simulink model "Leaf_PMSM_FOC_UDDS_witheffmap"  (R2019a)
settings: Solver=VariableStepAuto  StartTime=0.0  StopTime=764  FixedStep=1e-3  MaxStep=1e-3  RelTol=1e-3
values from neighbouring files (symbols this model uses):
  B = 0    [PMSM_EV_init_v2.m]    (also in Leaf_Initialization.m; Tesla_Initialization.m)
  Eoff = 201e-6    (= 0.000201)    [DeviceParam.m]
  Eoff_diode = 1.4e-3    (= 0.0014)    [DeviceParam.m]
  Eoff_Si = 2.15e-3    (= 0.00215)    [DeviceParam.m]
  Eon = 252e-6    (= 0.000252)    [DeviceParam.m]
  Eon_Si = 1.2e-3    (= 0.0012)    [DeviceParam.m]
  fs = 10000    [PMSM_EV_init_v2.m]    (also in Leaf_Initialization.m; Tesla_Initialization.m)
  I_DS_data = [-36 36 62]    [DeviceParam.m]
  IC_data = [0 30 60]    [DeviceParam.m]
  Inom = 75    [DeviceParam.m]    (also in Iqbal Husain - Example12_1.m = Psm/VsmNom)
  J = 0.3    [PMSM_EV_init_v2.m]    (also in Leaf_Initialization.m; Tesla_Initialization.m)
  Leaf_id_axis = [-2.296328E+02	-2.041181E+02	-1.786033E+02	-1.530886E+02	-1.275738E+02	-1.020590E+02	-7.654428E+01	-5.102952E+01	-2.551476E+01	+0.000000E+00]    [Leaf_Param.m]    (also in Leaf_Initialization.m)
  Leaf_iq_axis = [+0.000000E+00	+2.551476E+01	+5.102952E+01	+7.654428E+01	+1.020590E+02	+1.275738E+02	+1.530886E+02	+1.786033E+02	+2.041181E+02	+2.296328E+02]    [Leaf_Param.m]    (also in Leaf_Initialization.m)
  Leaf_Ld = [+4.562516E-04	+4.676675E-04	+4.893199E-04	+5.037353E-04	+5.104223E-04	+5.166612E-04	+5.237499E-04	+5.295159E-04	+5.345150E-04	+5.371060E-04    [Leaf_Param.m]    (also in Leaf_Initialization.m)
  Leaf_Lq = [+1.028048E-03	+1.047482E-03	+1.072792E-03	+1.100303E-03	+1.125549E-03	+1.152180E-03	+1.181188E-03	+1.211466E-03	+1.243133E-03	+1.273628E-03    [Leaf_Param.m]    (also in Leaf_Initialization.m)
  Leaf_omega_axis = [+0.000000E+00	+3.935365E+01	+7.870730E+01	+1.180610E+02	+1.574146E+02	+1.967683E+02	+2.361219E+02	+2.754756E+02	+3.857216E+02	+4.959676E+02	+6.062136E+02	+7.164596E+02	+8.267056E+02	+9.369516E+02	+1.047198E+03]    [Leaf_Param.m]    (also in Leaf_Initialization.m)
  Leaf_phid = [-4.199708E-02	-2.553401E-02	-8.247090E-03	+9.778563E-03	+2.810579E-02	+4.661402E-02	+6.539149E-02	+8.441129E-02	+1.036049E-01	+1.229854E-01    [Leaf_Param.m]    (also in Leaf_Initialization.m)
  Leaf_phiq = [-1.952292E-05	-3.396145E-06	+2.962394E-07	-2.077424E-05	-3.654397E-05	-1.649631E-05	+3.339687E-05	+4.306712E-05	+9.669480E-06	-2.373166E-05    [Leaf_Param.m]    (also in Leaf_Initialization.m)
  Leaf_T = [-3.804040E-02	-5.882121E-03	+4.489506E-04	-2.698573E-02	-3.955883E-02	-1.428580E-02	+2.169126E-02	+1.864805E-02	+2.093441E-03	+0.000000E+00    [Leaf_Param.m]    (also in Leaf_Initialization.m)
  Leaf_torque_axis = [+0.000000E+00	+1.167089E+01	+2.334179E+01	+3.501268E+01	+4.668357E+01	+5.835446E+01	+7.002536E+01	+7.910792E+01	+9.076234E+01	+1.063042E+02	+1.281510E+02	+1.612785E+02	+2.121831E+02	+2.805757E+02]    [Leaf_Param.m]    (also in Leaf_Initialization.m)
  P = 8    [PMSM_EV_init_v2.m]    (also in Iqbal Husain - Example12_1.m = V.*I; Leaf_Initialization.m; Tesla_Initialization.m)
  Rd_IGBT = (1.4-0.9)/(60-15)    (= 0.0111111111111)    [DeviceParam.m]
  RDS_on_data = [25e-3 27e-3 28e-3]    [DeviceParam.m]
  Rs = 0.046    [PMSM_EV_init_v2.m]    (also in Leaf_Initialization.m; Tesla_Initialization.m)
  Speed = [+0.000000E+00	+6.054730E+02	+1.210946E+03	+1.816419E+03	+2.421892E+03	+3.027365E+03	+3.632838E+03	+4.238311E+03	+5.775695E+03	+7.313079E+03	+8.850463E+03	+1.038785E+04	+1.192523E+04	+1.346262E+04	+1.500000E+04]    [PMSM_EV_init_v2.m]
  Torque = [+0.000000E+00	+7.333624E+00	+1.466725E+01	+2.200087E+01	+2.933450E+01	+3.666812E+01	+4.400174E+01	+5.043561E+01	+5.870849E+01	+6.980054E+01	+8.566293E+01	+1.107686E+02	+1.535327E+02	+2.089386E+02]    [PMSM_EV_init_v2.m]
  Vbatt = Vdc    (= 375)    [PMSM_EV_init_v2.m]    (also in Leaf_Initialization.m; Tesla_Initialization.m)
  VCE_data = [0 1.1 1.45]    [DeviceParam.m]
  Vd_IGBT = 1.5    [DeviceParam.m]
  Vdc = 375    [PMSM_EV_init_v2.m]    (also in Leaf_Initialization.m; Tesla_Initialization.m)
  Vnom = 300    [DeviceParam.m]
undefined symbols (not defined in the file or in its folder): A1, B1370, B766, HEV_Param, plecs
libraries: fl_lib x18, nesl_utility x9, sdl_lib x4, powerlib_meascontrol x3
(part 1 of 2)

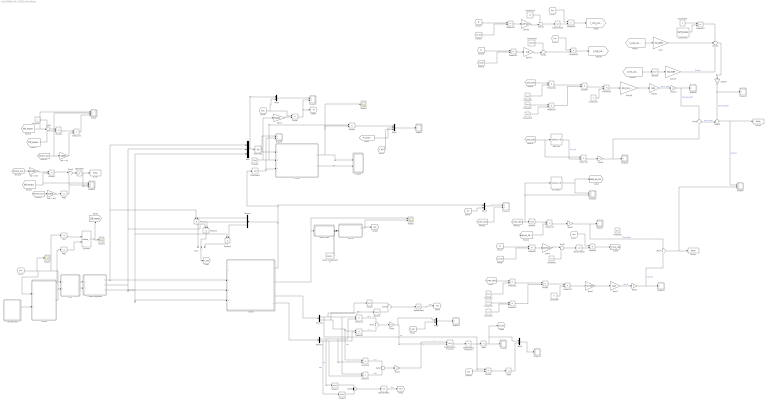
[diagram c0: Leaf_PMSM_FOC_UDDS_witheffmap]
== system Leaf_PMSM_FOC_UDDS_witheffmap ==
  Abs{,1..4} (5 alike) : Abs
  Circuit : Subsystem  LoadFcn=plecs('sl', 200);  InitFcn=plecs('sl', 214);  StartFcn=plecs('sl', 208);  StopFcn=plecs('sl', 209);  mask(PlecsCircuit){PLECSData=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}
      mask prompts: PLECSData "PLECS Data (Do not delete or modify!)"
      mask init:
      | % PLACE CUSTOM INITIALIZATIONS ABOVE
      | % DO NOT REMOVE
      | plecs('sl', 215);
      | % DO NOT REMOVE
  Constant : Constant  Value=Vbatt
  Constant1 : Constant  Value=1/8
  Constant10 : Constant  Value=Inom
  Constant11 : Constant  Value=fs
  Constant12 : Constant  Value=1/8
  Constant13 : Constant  Value=1/(2*pi)
  Constant14 : Constant  Value=fs
  Constant15 : Constant  Value=Eoff_diode
  Constant2 : Constant  Commented=on  Value=30e-3
  Constant3 : Constant  Value=Vbatt
  Constant4 : Constant  Value=Vnom
  Constant5 : Constant  Value=Inom
  Constant6 : Constant  Value=fs
  Constant7 : Constant
  Constant8 : Constant  Value=Vbatt
  Constant9 : Constant  Value=Vnom
  Control : Subsystem
  Current Regulator : Subsystem
  Currents : Subsystem  LoadFcn=plecs('sl', 300);  InitFcn=plecs('sl', 314);  StartFcn=plecs('sl', 308);  StopFcn=plecs('sl', 309);  mask{Settings=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}
      mask init:
      | plecs('sl', 315);
  Demux : Demux  Outputs=3
  Demux1 : Demux  Outputs=2
  Demux2 : Demux  Outputs=2
  Divide{,1..5} (6 alike) : Product  Inputs=*/
  FOC : Subsystem
  Gain : Gain  Gain=Vd_IGBT
  Gain1 : Gain  Gain=1.5
  Gain10 : Gain  Gain=Eon_Si+Eoff_Si
  Gain11 : Gain  Gain=1/pi
  Gain{5,8..9,12,16} (5 alike) : Gain  Gain=6
  Gain13 : Gain  Gain=1/(3*pi)
  Gain14 : Gain  Gain=1/8
  Gain15 : Gain  Gain=Rd_IGBT
  Gain2 : Gain  Gain=1.5
  Gain3 : Gain  Gain=1/sqrt(3)
  Gain4 : Gain  Gain=1/(3*pi)
  Gain6 : Gain  Gain=Eon+Eoff
  Gain7 : Gain  Gain=1/pi
  IGBT Vce : Lookup_n-D  NumberOfTableDimensions=1  BreakpointsForDimension1=IC_data  Table=VCE_data  InternalRulePriority=Speed  RndMeth=Simplest
  Iq_camry : Lookup_n-D  BreakpointsForDimension1=Leaf_omega_axis  BreakpointsForDimension2=Leaf_torque_axis  Table=Leaf_Eff'  InternalRulePriority=Speed  RndMeth=Simplest
  Kph demand : Subsystem
  Motor Shaft : Subsystem
  Mux : Mux  Inputs=3
  Mux1 : Mux  Inputs=3
  Mux{2..5} (4 alike) : Mux  Inputs=2
  PMSM : Subsystem
  Product{,1..23} (24 alike) : Product
  Saturation : Saturate  UpperLimit=10e3  LowerLimit=0
  Scope : Subsystem  LoadFcn=plecs('sl', 300);  InitFcn=plecs('sl', 314);  StartFcn=plecs('sl', 308);  StopFcn=plecs('sl', 309);  mask{Settings=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}
      mask init:
      | plecs('sl', 315);
  Scope1 : Scope
  Scope10 : Subsystem  LoadFcn=plecs('sl', 300);  InitFcn=plecs('sl', 314);  StartFcn=plecs('sl', 308);  StopFcn=plecs('sl', 309);  mask{Settings=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}
      mask init:
      | plecs('sl', 315);
  Scope11 : Subsystem  LoadFcn=plecs('sl', 300);  InitFcn=plecs('sl', 314);  StartFcn=plecs('sl', 308);  StopFcn=plecs('sl', 309);  mask{Settings=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}
      mask init:
      | plecs('sl', 315);
  Scope12 : Subsystem  LoadFcn=plecs('sl', 300);  InitFcn=plecs('sl', 314);  StartFcn=plecs('sl', 308);  StopFcn=plecs('sl', 309);  mask{Settings=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}
      mask init:
      | plecs('sl', 315);
  Scope13 : Subsystem  LoadFcn=plecs('sl', 300);  InitFcn=plecs('sl', 314);  StartFcn=plecs('sl', 308);  StopFcn=plecs('sl', 309);  mask{Settings=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}
      mask init:
      | plecs('sl', 315);
  Scope14 : Subsystem  LoadFcn=plecs('sl', 300);  InitFcn=plecs('sl', 314);  StartFcn=plecs('sl', 308);  StopFcn=plecs('sl', 309);  mask{Settings=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}
      mask init:
      | plecs('sl', 315);
  Scope15 : Subsystem  LoadFcn=plecs('sl', 300);  InitFcn=plecs('sl', 314);  StartFcn=plecs('sl', 308);  StopFcn=plecs('sl', 309);  mask{Settings=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}
      mask init:
      | plecs('sl', 315);
  Scope16 : Subsystem  LoadFcn=plecs('sl', 300);  InitFcn=plecs('sl', 314);  StartFcn=plecs('sl', 308);  StopFcn=plecs('sl', 309);  mask{Settings=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}
      mask init:
      | plecs('sl', 315);
  Scope17 : Subsystem  LoadFcn=plecs('sl', 300);  InitFcn=plecs('sl', 314);  StartFcn=plecs('sl', 308);  StopFcn=plecs('sl', 309);  mask{Settings=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}
      mask init:
      | plecs('sl', 315);
  Scope18 : Subsystem  LoadFcn=plecs('sl', 300);  InitFcn=plecs('sl', 314);  StartFcn=plecs('sl', 308);  StopFcn=plecs('sl', 309);  mask{Settings=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}
      mask init:
      | plecs('sl', 315);
  Scope19 : Subsystem  LoadFcn=plecs('sl', 300);  InitFcn=plecs('sl', 314);  StartFcn=plecs('sl', 308);  StopFcn=plecs('sl', 309);  mask{Settings=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}
      mask init:
      | plecs('sl', 315);
  Scope2 : Scope  NumInputPorts=2
  Scope3 : Scope
  Scope4 : Subsystem  LoadFcn=plecs('sl', 300);  InitFcn=plecs('sl', 314);  StartFcn=plecs('sl', 308);  StopFcn=plecs('sl', 309);  mask{Settings=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}
      mask init:
      | plecs('sl', 315);
  Scope5 : Subsystem  LoadFcn=plecs('sl', 300);  InitFcn=plecs('sl', 314);  StartFcn=plecs('sl', 308);  StopFcn=plecs('sl', 309);  mask{Settings=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}
      mask init:
      | plecs('sl', 315);
  Scope6 : Subsystem  LoadFcn=plecs('sl', 300);  InitFcn=plecs('sl', 314);  StartFcn=plecs('sl', 308);  StopFcn=plecs('sl', 309);  mask{Settings=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}
      mask init:
      | plecs('sl', 315);
  Scope7 : Scope
  Scope8 : Subsystem  LoadFcn=plecs('sl', 300);  InitFcn=plecs('sl', 314);  StartFcn=plecs('sl', 308);  StopFcn=plecs('sl', 309);  mask{Settings=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}
      mask init:
      | plecs('sl', 315);
  Scope9 : Subsystem  LoadFcn=plecs('sl', 300);  InitFcn=plecs('sl', 314);  StartFcn=plecs('sl', 308);  StopFcn=plecs('sl', 309);  mask{Settings=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}
      mask init:
      | plecs('sl', 315);
  SiC RdsOn : Lookup_n-D  NumberOfTableDimensions=1  BreakpointsForDimension1=I_DS_data  Table=RDS_on_data  InternalRulePriority=Speed  RndMeth=Simplest
  Solver Configuration : nesl_utility/Solver Configuration  PhysicalDomain=network_engine_domain  SubClassName=solver  LeftPortType=input  RightPortType=generic  Tones=[]  Harmonics=[]  SimulateNoise=off  Profile=off  UseLocalSampling=off  EnableSwitchedLinearOptims=on  FrequencyDomain=off  UseCCode=off  RelTol=0.001  AbsTol=1e-06  MinStep=1e-09  ToWorkspace=off  RevertToSquareIcSolve=off  NumHomotopyIterations=100  PhasorMode=off  PhasorModeNumHarmonics=1  DoDC=off  ResidualTolerance=1e-09  UseLocalSolver=off  LocalSolverChoice=NE_BACKWARD_EULER_ADVANCER  LocalSolverSampleTime=0.001  DoFixedCost=off  MaxNonlinIter=3  MaxModeIter=2  LinearAlgebra=auto  EquationFormulation=NE_TIME_EF  DelaysMemoryBudget=1024  AutomaticFiltering=on  FilteringTimeConstant=0.001  PartitionStorageMethod=AS_NEEDED  PartitionMemoryBudget=1024  PartitionMethod=FAST
  Square{,1..5} (6 alike) : Math  Operator=square
  Square Root{,1..3} (4 alike) : Sqrt
  Sum : Sum  Inputs=3
  Sum{1,3..4,7,9} (5 alike) : Sum  Inputs=+|+
  Sum10 : Sum  Inputs=+-|
  Sum11 : Sum  Inputs=+-|
  Sum12 : Sum  Inputs=+++
  Sum13 : Sum  Inputs=++|
  Sum2 : Sum  Inputs=+|-
  Sum5 : Sum  Inputs=|++
  Sum6 : Sum  Inputs=+-|
  Sum8 : Sum  Inputs=|+-
  To File : ToFile  Filename=PLoss_motor.mat  MatrixName=PLoss_motor  SaveFormat=Timeseries
  To File1 : ToFile  Filename=PLoss_inv.mat  MatrixName=PLoss_inv  SaveFormat=Timeseries
  To File2 : ToFile  Filename=PLoss_inv_Si.mat  MatrixName=PLoss_inv_Si  SaveFormat=Timeseries
  Trigonometric Function : Trigonometry  Operator=atan2
  Trigonometric Function1 : Trigonometry  Operator=cos
  Unit Delay : UnitDelay  SampleTime=-1  HasFrameUpgradeWarning=on
  Unit Delay1 : UnitDelay  SampleTime=-1  HasFrameUpgradeWarning=on
  Vehicle : Subsystem
  "kW -> W" : Gain  Gain=1000
  "kW -> W1" : Gain  Gain=1000
  "kW -> W2" : Gain  Gain=1000
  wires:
  [wm] -> Scope1/1, Abs/1, FOC/1(Speed), Control/1("rad/s ")
  FOC/2(Id_ref) -> Current Regulator/2(id_ref)
  PMSM/3(Torque (Nm)) -> Scope2/1, Motor Shaft/1(In1)
  Control/1(Mot_TReq) -> Abs1/1, FOC/2(Torque)
  Kph demand/1(Acc) -> Control/2(Acc)
  FOC/1(Iq_ref) -> Current Regulator/1(iq_ref)
  Vehicle/1(VehSpd) -> Scope2/2, [kph]
  Abs/1 -> Iq_camry/1
  Abs1/1 -> Iq_camry/2
  Iq_camry/1 -> Scope3/1, [Eff_motor]
  Mux4/1 -> Scope10/1(1)
  Product/1 -> Mux1/1
  [P_VSI] -> Mux1/3
  Divide/1 -> [M], Scope10/2(2)
  [Vsm] -> Mux4/2, Divide/1
  Circuit/1(I_batt) -> Scope7/1, Product/2, Scope5/1(1)
  Gain3/1 -> Divide/2
  Unit Delay1/1 -> Circuit/3(Iabc_ref), Scope4/2(2)
  Unit Delay/1 -> Circuit/1(m), Scope4/1(1)
  Circuit/2(I_abc) -> Scope5/2(2)
  [P_motor] -> Mux1/2
  Constant/1 -> Gain3/1, Product/1, Circuit/2(Vbatt_ref)
  Mux1/1 -> Scope6/1(1)
  Mux/1 -> Mux4/1, Unit Delay/1
  Gain5/1 -> Sum7/1, Scope9/1(1)  "Pcond,total"
  [Rds_on_calc] -> Product10/2
  Product10/1 -> Gain5/1
  Product8/1 -> Gain4/1
  [I_rms_calc] -> Scope13/2(2), SiC RdsOn/1, Square4/1
  Product9/1 -> [I_rms_calc]
  Gain4/1 -> Sum5/1
  [I_rms_calc] -> Currents/2(2)
  [Ism] -> Product9/1
  Constant1/1 -> Sum5/2
  [M] -> Product8/1
  Square Root2/1 -> Product9/2
  [cos_phi] -> Product8/2
  [Ism] -> Mux3/2
  Mux3/1 -> Currents/1(1)
  Sum5/1 -> Square Root2/1
  Square4/1 -> Product10/1
  Sum1/1 -> Gain1/1
  Abs2/1 -> Mux5/1, [cos_phi], Scope8/1(1)
  [P_VSI] -> Mux2/2
  Product5/1 -> Sum1/2  "vdid"
  Product4/1 -> Sum1/1  "vqiq"
  Square/1 -> Sum3/1
  Square3/1 -> Sum4/2
  Sum4/1 -> Square Root1/1
  Square Root1/1 -> [Vsm]  "Ism"
  Mux2/1 -> Scope11/1(1)
  Sum3/1 -> Square Root/1
  Square1/1 -> Sum3/2
  Gain1/1 -> Mux2/1, Trigonometric Function/2  "P"
  Square Root/1 -> [Ism]  "Ism"
  Trigonometric Function1/1 -> Abs2/1
  Demux2/2 -> Square3/1, Product7/2, Product5/2  "vdm"
  Trigonometric Function/1 -> Trigonometric Function1/1
  Product6/1 -> Sum2/1  "vqid"
  Sum2/1 -> Gain2/1
  Square2/1 -> Sum4/1
  Demux2/1 -> Square2/1, Product6/2, Product4/2  "vqm"
  Demux1/1 -> Divide5/1, Square/1, Product7/1, Product4/1  "iqm"
  Gain2/1 -> Trigonometric Function/1  "Q"
  Demux1/2 -> Square1/1, Product6/1, Product5/1  "idm"
  PMSM/6(vqd,m) -> Demux2/1
  PMSM/5(iqd,m) -> Demux1/1
  Product7/1 -> Sum2/2  "vdiq"
  Demux/3 -> Product1/2
  Current Regulator/3(Vc) -> PMSM/4(Vc), Product1/1, Mux/3
  Product1/1 -> Sum/3
  Product2/1 -> Sum/2
  Demux/1 -> Product3/2
  Demux/2 -> Product2/2
  Sum/1 -> [P_VSI]
  Product3/1 -> Sum/1
  Current Regulator/2(Vb) -> PMSM/3(Vb), Mux/2, Product2/1
  PMSM/1(iabc) -> Unit Delay1/1, Mux3/1, Demux/1
  Current Regulator/1(Va) -> PMSM/2(Va), Product3/1, Mux/1
  [I_rms_calc] -> Product11/1
  Constant3/1 -> Product11/2
  Product11/1 -> Divide1/1
  Constant4/1 -> Product12/1
  Constant5/1 -> Product12/2
  Product12/1 -> Divide1/2
  Divide1/1 -> Product13/1
  Constant6/1 -> Product13/2
  Product13/1 -> Gain6/1
  Gain6/1 -> Gain7/1
  Gain7/1 -> Gain8/1  "Psw,Q"
  Gain8/1 -> Sum7/2, Scope12/1(1)  "Psw,total"
  SiC RdsOn/1 -> [Rds_on_calc], Scope13/1(1)
  [Eff_motor] -> Scope/1(1), Sum6/2
  Constant7/1 -> Sum6/1
  Sum6/1 -> Divide2/1
  [Eff_motor] -> Divide2/2
  Divide2/1 -> Product14/1
  [Pmotor_out] -> Scope/2(2), "kW -> W"/1
  Product14/1 -> Scope/3(3)
  Sum7/1 -> Scope17/2(2), To File1/1
  "kW -> W"/1 -> Product14/2
  [Pmotor_out] -> "kW -> W1"/1
  "kW -> W1"/1 -> Divide3/1
  [Eff_motor] -> Divide3/2, Scope14/1(1)
  Divide3/1 -> Sum8/1
  Sum8/1 -> Saturation/1
  Abs3/1 -> Scope14/2(2), Sum8/2
  Saturation/1 -> Scope14/3(3), To File/1
  [Pmotor_out] -> "kW -> W2"/1
  "kW -> W2"/1 -> Abs3/1
  IGBT Vce/1 -> Product15/2  "Vce_calc"
  [I_rms_calc] -> Product15/1, IGBT Vce/1
  Gain9/1 -> Sum9/2, Scope15/1(1)
  Product15/1 -> Gain9/1
  Gain11/1 -> Gain12/1  "Psw,Q_IGBT"
  Divide4/1 -> Product18/1
  Gain10/1 -> Gain11/1
  Product17/1 -> Divide4/2
  Constant8/1 -> Product16/2
  Constant9/1 -> Product17/1
  Product16/1 -> Divide4/1
  [I_rms_calc] -> Product16/1
  Constant10/1 -> Product17/2
  Product18/1 -> Gain10/1
  Constant11/1 -> Product18/2
  Gain12/1 -> Sum9/1, Scope16/1(1)  "Psw,total_IGBT"
  Sum10/1 -> Square Root3/1
  Square Root3/1 -> Product20/2
  [M] -> Product19/1
  Product19/1 -> Gain13/1
  Product20/1 -> [I_rms_calc_diode]
  [Ism] -> Product20/1
  [cos_phi] -> Product19/2
  Gain13/1 -> Sum10/2
  Constant12/1 -> Sum10/1
  Gain14/1 -> Sum11/2
  Constant13/1 -> Sum11/1
  [cos_phi] -> Product21/2
  [Ism] -> Product22/1
  Product22/1 -> [I_avg_calc_diode]
  Sum11/1 -> Product22/2
  [M] -> Product21/1
  Product21/1 -> Gain14/1
  [I_avg_calc_diode] -> Gain/1
  [I_rms_calc_diode] -> Square5/1
  Square5/1 -> Gain15/1
  Constant14/1 -> Product23/1
  Constant15/1 -> Product23/2
  Product23/1 -> Sum12/1
  Gain15/1 -> Sum12/3  "P_diode"
  Gain/1 -> Sum12/2
  Sum9/1 -> Sum13/2  "Ptotal_IGBT"
  Sum13/1 -> Scope17/1(1), To File2/1  "Ptotal_Si"
  Gain16/1 -> Scope18/1(1), Sum13/1  "Psw,total_IGBT"
  Sum12/1 -> Gain16/1
  Mux5/1 -> Scope19/1(1)
  [Ism] -> Divide5/2
  Divide5/1 -> Abs4/1
  Abs4/1 -> Mux5/2
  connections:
  Motor Shaft/RConn1 -- Vehicle/LConn1 -- Solver Configuration/RConn1

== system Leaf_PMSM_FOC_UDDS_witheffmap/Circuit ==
  m : Inport  PortDimensions=3
  Vbatt_ref : Inport  Port=2  PortDimensions=1
  Iabc_ref : Inport  Port=3  PortDimensions=3
  " GateMux " : Ground
  " Iabc_ref " : DataTypeConversion
  " InputMux " : Mux  Inputs=[ 3 1 3 ]
  " OutputDemux " : Demux  Outputs=[ 1 3 ]
  " ProbeDemux " : Terminator
  " S-Function " : S-Function  FunctionName=plecs  SFunctionDeploymentMode=off  EnableBusSupport=off
  " Vbatt_ref " : DataTypeConversion
  " m " : DataTypeConversion
  I_batt : Outport  PortDimensions=1
  I_abc : Outport  Port=2  PortDimensions=3
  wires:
  " InputMux "/1 -> " S-Function "/1
  " GateMux "/1 -> " S-Function "/2
  " S-Function "/1 -> " OutputDemux "/1
  " S-Function "/2 -> " ProbeDemux "/1
  m/1 -> " m "/1
  " m "/1 -> " InputMux "/1
  Vbatt_ref/1 -> " Vbatt_ref "/1
  " Vbatt_ref "/1 -> " InputMux "/2
  Iabc_ref/1 -> " Iabc_ref "/1
  " Iabc_ref "/1 -> " InputMux "/3
  " OutputDemux "/1 -> I_batt/1
  " OutputDemux "/2 -> I_abc/1

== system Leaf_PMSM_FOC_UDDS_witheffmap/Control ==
  "rad/s " : Inport
  Acc : Inport  Port=2
  Constant : Constant
  Convert acceleration demand to motor speed demand. : Lookup  InputValues=[0 30]  Table=[0 10000]
  Gain : Gain  Gain=60/(2*pi)
  Motor Controller : Subsystem
  Scope : Scope
  Subsystem : Subsystem
  Subsystem1 : Subsystem
  Mot_TReq : Outport
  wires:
  Acc/1 -> Subsystem1/1(In1)
  Convert acceleration demand to motor speed demand./1 -> Subsystem/1(In1)
  Motor Controller/1(M_Trq_Dem) -> Mot_TReq/1
  Constant/1 -> [Mot_Enable]
  Subsystem/1(Motor_RPM_Dem) -> Scope/1, Motor Controller/2(Mot_RPM_Dem)
  [Mot_Enable] -> Motor Controller/1(Mot_Enable)
  "rad/s "/1 -> Gain/1
  Subsystem1/1(Accel) -> Convert acceleration demand to motor speed demand./1
  Gain/1 -> Motor Controller/3(Mot_RPM)

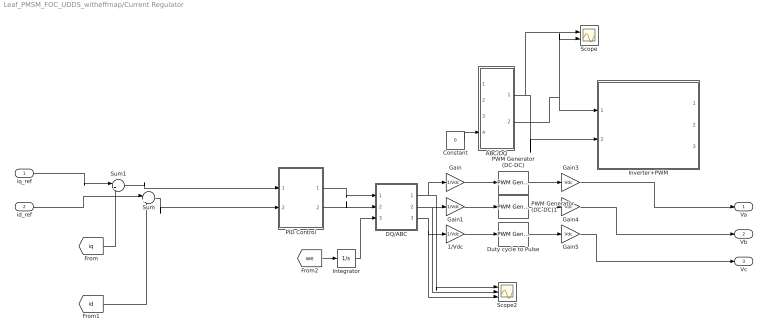
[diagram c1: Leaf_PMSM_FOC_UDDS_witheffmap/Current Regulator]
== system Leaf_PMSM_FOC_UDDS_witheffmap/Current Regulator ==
  iq_ref : Inport
  id_ref : Inport  Port=2
  1/Vdc : Gain  Commented=through  Gain=1/Vdc
  ABC/DQ : Subsystem  Commented=on
  Constant : Constant  Commented=on  Value=0
  DQ/ABC : Subsystem
  Duty cycle to Pulse : powerlib_meascontrol/Pulse & Signal Generators/PWM Generator (DC-DC)  Commented=through  Fsw=50  Ts=1e-4
  Gain : Gain  Commented=through  Gain=1/Vdc
  Gain1 : Gain  Commented=through  Gain=1/Vdc
  Gain3 : Gain  Commented=through  Gain=Vdc
  Gain4 : Gain  Commented=through  Gain=Vdc
  Gain5 : Gain  Commented=through  Gain=Vdc
  Integrator : Integrator
  Inverter+PWM : Subsystem  Commented=on
  PID Control : Subsystem
  PWM Generator (DC-DC) : powerlib_meascontrol/Pulse & Signal Generators/PWM Generator (DC-DC)  Commented=through  Fsw=50  Ts=1e-4
  PWM Generator (DC-DC)1 : powerlib_meascontrol/Pulse & Signal Generators/PWM Generator (DC-DC)  Commented=through  Fsw=50  Ts=1e-4
  Scope : Scope  NumInputPorts=2
  Scope2 : Scope  NumInputPorts=3
  Sum : Sum  Inputs=|+-
  Sum1 : Sum  Inputs=|+-
  Va : Outport
  Vb : Outport  Port=2
  Vc : Outport  Port=3
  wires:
  [iq] -> Sum1/2
  [id] -> Sum/2
  PID Control/1(Out1) -> DQ/ABC/1(Vq)
  Sum/1 -> PID Control/2(In3)
  PID Control/2(Out2) -> DQ/ABC/2(Vd)
  id_ref/1 -> Sum/1
  [we] -> Integrator/1
  iq_ref/1 -> Sum1/1
  Integrator/1 -> DQ/ABC/3(theta_rf)
  Sum1/1 -> PID Control/1(In1)
  Inverter+PWM/3(Vc) -> ?
  ABC/DQ/1(d) -> Scope/1, Inverter+PWM/2(vd)
  Inverter+PWM/1(Va) -> ?
  Constant/1 -> ABC/DQ/4(omega_rf)
  ABC/DQ/2("q ") -> Scope/2, Inverter+PWM/1(vq)
  ? -> ABC/DQ/2(Vb)
  ? -> ABC/DQ/3(Vc)
  Inverter+PWM/2(Vb) -> ?
  ? -> ABC/DQ/1(Va)
  DQ/ABC/1(Va) -> Scope2/1, Gain/1
  DQ/ABC/2("Vb ") -> Scope2/2, Gain1/1
  DQ/ABC/3("Vc ") -> Scope2/3, 1/Vdc/1
  Gain/1 -> PWM Generator (DC-DC)/1
  Gain1/1 -> PWM Generator (DC-DC)1/1
  1/Vdc/1 -> Duty cycle to Pulse/1
  PWM Generator (DC-DC)/1 -> Gain3/1
  PWM Generator (DC-DC)1/1 -> Gain4/1
  Duty cycle to Pulse/1 -> Gain5/1
  Gain3/1 -> Va/1
  Gain4/1 -> Vb/1
  Gain5/1 -> Vc/1

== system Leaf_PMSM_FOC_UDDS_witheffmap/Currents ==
  1 : Inport
  2 : Inport  Port=2
  " 1 " : DataTypeConversion
  " 2 " : DataTypeConversion
  " InputMux " : Mux  Inputs=2
  " S-Function " : S-Function  FunctionName=plecs  SFunctionDeploymentMode=off  EnableBusSupport=off
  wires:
  " InputMux "/1 -> " S-Function "/1
  1/1 -> " 1 "/1
  " 1 "/1 -> " InputMux "/1
  2/1 -> " 2 "/1
  " 2 "/1 -> " InputMux "/2

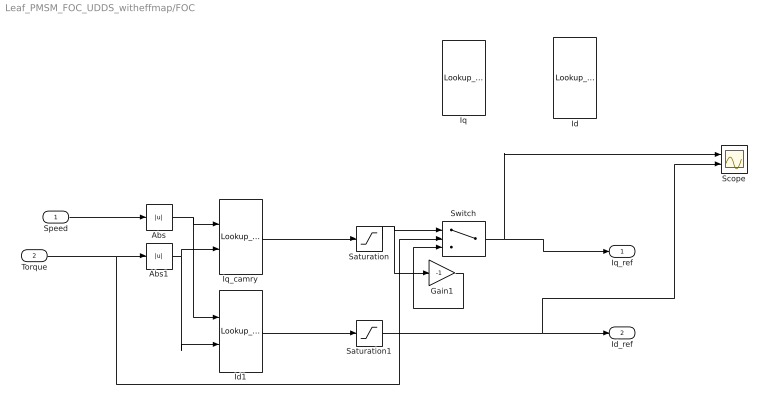
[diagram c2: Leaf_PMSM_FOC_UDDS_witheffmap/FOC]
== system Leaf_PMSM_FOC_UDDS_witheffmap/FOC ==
  Speed : Inport
  Torque : Inport  Port=2
  Abs : Abs
  Abs1 : Abs
  Gain1 : Gain  Gain=-1
  Id : Lookup_n-D  Commented=on  BreakpointsForDimension1=Speed  BreakpointsForDimension2=Torque  Table=Id_C'  InternalRulePriority=Speed  RndMeth=Simplest
  Id1 : Lookup_n-D  BreakpointsForDimension1=Leaf_omega_axis  BreakpointsForDimension2=Leaf_torque_axis  Table=Leaf_Id'  InternalRulePriority=Speed  RndMeth=Simplest
  Iq : Lookup_n-D  Commented=on  BreakpointsForDimension1=Speed  BreakpointsForDimension2=Torque  Table=Iq_C'  InternalRulePriority=Speed  RndMeth=Simplest
  Iq_camry : Lookup_n-D  BreakpointsForDimension1=Leaf_omega_axis  BreakpointsForDimension2=Leaf_torque_axis  Table=Leaf_Iq'  InternalRulePriority=Speed  RndMeth=Simplest
  Saturation : Saturate  UpperLimit=300  LowerLimit=-300
  Saturation1 : Saturate  UpperLimit=300  LowerLimit=-300
  Scope : Scope  NumInputPorts=2
  Switch : Switch  Criteria=u2 > Threshold
  Iq_ref : Outport
  Id_ref : Outport  Port=2
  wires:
  Abs/1 -> Id1/1, Iq_camry/1
  Abs1/1 -> Id1/2, Iq_camry/2
  Speed/1 -> Abs/1
  Id1/1 -> Saturation1/1
  Switch/1 -> Scope/1, Iq_ref/1
  Torque/1 -> Switch/2, Abs1/1
  Gain1/1 -> Switch/3
  Saturation/1 -> Gain1/1, Switch/1
  Saturation1/1 -> Scope/2, Id_ref/1
  Iq_camry/1 -> Saturation/1

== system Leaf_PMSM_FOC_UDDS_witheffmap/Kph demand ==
  From Spreadsheet1 : FromSpreadsheet  FileName=Highway_cycle.xlsx  Range=A1:B766  ExtrapolationBeforeFirstDataPoint=Hold first value
  From Spreadsheet2 : FromSpreadsheet  FileName=Highway_cycle.xlsx  Range=A1:B766  ExtrapolationBeforeFirstDataPoint=Hold first value
  From Spreadsheet3 : FromSpreadsheet  Commented=on  FileName=LA4_Cycle.xlsx  Range=A1:B1370  ExtrapolationBeforeFirstDataPoint=Hold first value
  Gain : Gain  Gain=1.6
  Gain1 : Gain  Gain=0.44704
  Gain2 : Gain  Gain=1/1600
  Integrator : Integrator
  Scope : Scope  NumInputPorts=2
  Scope1 : Scope
  Vehicle Speed Controller : Subsystem
  Acc : Outport
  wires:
  From Spreadsheet1/1 -> Gain/1
  [kph] -> Scope/2, Vehicle Speed Controller/2(Veh Spd)
  Gain/1 -> Scope/1, Vehicle Speed Controller/1(Ref Spd)
  Vehicle Speed Controller/1(Acc) -> Acc/1
  From Spreadsheet2/1 -> Gain1/1
  Gain1/1 -> Integrator/1
  Integrator/1 -> Gain2/1
  Gain2/1 -> Scope1/1

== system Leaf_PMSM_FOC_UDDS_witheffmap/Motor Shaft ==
  In1 : Inport
  Ideal Rotational Motion Sensor : fl_lib/Mechanical/Mechanical Sensors/Ideal Rotational Motion Sensor  offset=0 rad
  Ideal Torque Source : fl_lib/Mechanical/Mechanical Sources/Ideal Torque Source
  Mechanical Rotational Reference : fl_lib/Mechanical/Rotational Elements/Mechanical Rotational Reference
  Mechanical Rotational Reference1 : fl_lib/Mechanical/Rotational Elements/Mechanical Rotational Reference
  PS-Simulink Converter : nesl_utility/PS-Simulink Converter  PhysicalDomain=network_engine_domain  SubClassName=ps_output  LeftPortType=input  RightPortType=output  PseudoPeriodic=off  Frequencies=[]  Unit=rad/s  AffineConversion=off
  Shaft Inertia : fl_lib/Mechanical/Rotational Elements/Inertia  inertia=HEV_Param.Motor.Shaft_Inertia kg*m^2  w_specify=on  w_priority=High  w=0 rad/s  w_nominal_specify=off  w_nominal_unit=rad/s  w_nominal_value=1  t_specify=off  t_priority=High  t=0 N*m  t_nominal_specify=off  t_nominal_unit=N*m  t_nominal_value=1
  Simulink-PS Converter : nesl_utility/Simulink-PS Converter  PhysicalDomain=network_engine_domain  SubClassName=ps_input  LeftPortType=input  RightPortType=output  PseudoPeriodic=off  Frequencies=[]  NoiseDistribution=none  NoiseParameters=[]  Unit=1  AffineConversion=off  FilteringAndDerivatives=zero  SimscapeFilterOrder=1  InputFilterTimeConstant=.001  UdotUserProvided=0
  Sh : PMIOPort  Side=Right
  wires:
  In1/1 -> Simulink-PS Converter/1
  PS-Simulink Converter/1 -> [wm]
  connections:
  Mechanical Rotational Reference1/LConn1 -- Ideal Torque Source/RConn2
  Ideal Torque Source/LConn1 -- Ideal Rotational Motion Sensor/LConn1 -- Shaft Inertia/LConn1 -- Sh/RConn1
  Simulink-PS Converter/RConn1 -- Ideal Torque Source/RConn1
  Mechanical Rotational Reference/LConn1 -- Ideal Rotational Motion Sensor/RConn1
  PS-Simulink Converter/LConn1 -- Ideal Rotational Motion Sensor/RConn2

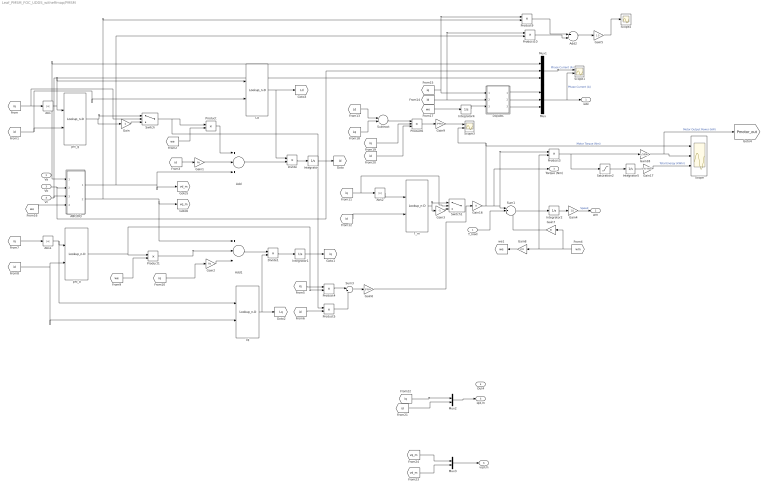
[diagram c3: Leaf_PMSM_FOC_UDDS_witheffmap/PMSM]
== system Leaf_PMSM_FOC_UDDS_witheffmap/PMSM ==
  T_load : Inport
  Va : Inport  Port=2
  Vb : Inport  Port=3
  Vc : Inport  Port=4
  ABC/DQ : Subsystem
  Abs : Abs
  Abs1 : Abs
  Abs2 : Abs
  Add : Sum  Inputs=+-+
  Add1 : Sum  Inputs=+--
  Add2 : Sum
  DQ/ABC : Subsystem
  Divide : Product  Inputs=/*
  Divide1 : Product  Inputs=*/
  Gain : Gain  Gain=-1
  Gain1 : Gain  Gain=Rs
  Gain16 : Gain
  Gain17 : Gain  Gain=2.77778e-7
  Gain18 : Gain  Gain=1/1000
  Gain2 : Gain  Gain=Rs
  Gain3 : Gain  Gain=-1
  Gain4 : Gain  Gain=1/J
  Gain5 : Gain  Gain=1.5
  Gain6 : Gain  Gain=3*P/4
  Gain7 : Gain  Gain=B
  Gain8 : Gain  Gain=P/2
  Gain9 : Gain  Gain=3*P/4
  Integrator{,1..2,4..5} (5 alike) : Integrator
  Ld : Lookup_n-D  BreakpointsForDimension1=Leaf_iq_axis  BreakpointsForDimension2=Leaf_id_axis  Table=Leaf_Ld  InternalRulePriority=Speed  RndMeth=Simplest
  Lq : Lookup_n-D  BreakpointsForDimension1=Leaf_iq_axis  BreakpointsForDimension2=Leaf_id_axis  Table=Leaf_Lq  InternalRulePriority=Speed  RndMeth=Simplest
  Mux : Mux  Inputs=3
  Mux1 : Mux  Inputs=3
  Mux2 : Mux  Inputs=2
  Mux3 : Mux  Inputs=2
  Product{,1,3..5,9..10} (7 alike) : Product
  Product6 : Product  Inputs=3
  Saturation2 : Saturate  UpperLimit=inf  LowerLimit=0
  Scope : Scope  NumInputPorts=3
  Scope1 : Scope  NumInputPorts=2
  Scope2 : Scope
  Scope3 : Scope  NumInputPorts=2
  Subtract : Sum  Inputs=+-
  Sum1 : Sum  Inputs=|+--
  Sum3 : Sum  Inputs=|+-
  Switch : Switch  Criteria=u2 > Threshold
  Switch1 : Switch  Criteria=u2 > Threshold
  T_m : Lookup_n-D  BreakpointsForDimension1=Leaf_iq_axis  BreakpointsForDimension2=Leaf_id_axis  Table=Leaf_T  ExtrapMethod=Clip  UseLastTableValue=on  InternalRulePriority=Speed  RndMeth=Simplest
  phi_d : Lookup_n-D  BreakpointsForDimension1=Leaf_iq_axis  BreakpointsForDimension2=Leaf_id_axis  Table=Leaf_phid  InternalRulePriority=Speed  RndMeth=Simplest
  phi_q : Lookup_n-D  BreakpointsForDimension1=Leaf_iq_axis  BreakpointsForDimension2=Leaf_id_axis  Table=Leaf_phiq  InternalRulePriority=Speed  RndMeth=Simplest
  iabc : Outport
  wm : Outport  Port=2
  Torque (Nm) : Outport  Port=3
  Out4 : Outport  Port=4
  iqd,m : Outport  Port=5
  vqd,m : Outport  Port=6
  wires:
  [iq] -> Abs1/1
  Divide1/1 -> Integrator1/1
  [we] -> ABC/DQ/4(omega_rf)
  T_m/1 -> Gain3/1, Switch1/1
  [id] -> Lq/2, phi_d/2
  [id] -> Ld/2, phi_q/2
  Vb/1 -> Mux1/2, ABC/DQ/2(Vb)
  Integrator4/1 -> DQ/ABC/3(theta_rf)
  [we] -> Integrator4/1
  [iq] -> Product9/1, DQ/ABC/1(Iq)
  Abs/1 -> Ld/1, phi_q/1
  Gain4/1 -> wm/1  "Speed"
  Divide/1 -> Integrator/1
  Add1/1 -> Divide1/1
  Gain1/1 -> Add/2
  [id] -> Product10/1, DQ/ABC/2(Id)
  Abs1/1 -> Lq/1, phi_d/1
  Integrator2/1 -> Gain4/1
  Ld/1 -> [Ld], Divide/1
  [we] -> Product/2
  phi_q/1 -> Gain/1, Switch/1
  Product/1 -> Add/1
  Integrator1/1 -> [iq]
  T_load/1 -> Sum1/2
  [iq] -> Switch/2, Abs/1
  Add/1 -> Divide/2
  Sum1/1 -> Integrator2/1
  Abs2/1 -> T_m/1
  [we] -> Product1/2
  Va/1 -> Mux1/1, ABC/DQ/1(Va)
  Integrator/1 -> [id]
  Gain/1 -> Switch/3
  Lq/1 -> [Lq], Divide1/2
  Mux/1 -> Scope1/2, iabc/1  "Phase Current (A)"
  Gain3/1 -> Switch1/3
  Gain2/1 -> Add1/3
  DQ/ABC/2("Ib ") -> Mux/2
  DQ/ABC/3("Ic ") -> Mux/3
  Gain7/1 -> Sum1/3
  Gain8/1 -> [we]
  [id] -> T_m/2
  Gain16/1 -> Torque (Nm)/1, Product3/1, Sum1/1, Scope/1, Scope3/2  "Motor Torque (Nm)"
  [iq] -> Abs2/1, Switch1/2
  Product3/1 -> Saturation2/1, Gain18/1
  Integrator5/1 -> Gain17/1
  Gain17/1 -> Scope/3  "Total Energy (kWhr)"
  Gain18/1 -> [Pmotor_out], Scope/2  "Motor Output Power (kW)"
  Saturation2/1 -> Integrator5/1
  Vc/1 -> Mux1/3, ABC/DQ/3(Vc)
  ABC/DQ/2("q ") -> Product9/2, [vq_m], Add1/1
  [id] -> Gain1/1
  ABC/DQ/1(d) -> Product10/2, [vd_m], Add/3
  [iq] -> Gain2/1
  DQ/ABC/1(Ia) -> Mux/1
  Mux1/1 -> Scope1/1  "Phase Current (A)"
  Product10/1 -> Add2/2
  Product9/1 -> Add2/1
  Add2/1 -> Gain5/1
  phi_d/1 -> Product4/2, Product1/1
  Product1/1 -> Add1/2
  Switch/1 -> Product5/1, Product/1
  [wm] -> Gain8/1, Product3/2, Gain7/1
  [iq] -> Product4/1
  Product4/1 -> Sum3/1
  [id] -> Product5/2
  Product5/1 -> Sum3/2
  Sum3/1 -> Gain6/1
  Gain5/1 -> Scope2/1
  [Ld] -> Subtract/1
  [Lq] -> Subtract/2
  Subtract/1 -> Product6/1
  [iq] -> Product6/2
  [id] -> Product6/3
  Product6/1 -> Gain9/1
  Gain9/1 -> Scope3/1
  Gain6/1 -> Gain16/1
  [vd_m] -> Mux3/2
  [vq_m] -> Mux3/1
  [iq] -> Mux2/1
  Mux2/1 -> iqd,m/1
  [id] -> Mux2/2
  Mux3/1 -> vqd,m/1

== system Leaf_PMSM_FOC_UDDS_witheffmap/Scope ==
  1 : Inport
  2 : Inport  Port=2
  3 : Inport  Port=3
  " 1 " : DataTypeConversion
  " 2 " : DataTypeConversion
  " 3 " : DataTypeConversion
  " InputMux " : Mux  Inputs=3
  " S-Function " : S-Function  FunctionName=plecs  SFunctionDeploymentMode=off  EnableBusSupport=off
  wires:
  " InputMux "/1 -> " S-Function "/1
  1/1 -> " 1 "/1
  " 1 "/1 -> " InputMux "/1
  2/1 -> " 2 "/1
  " 2 "/1 -> " InputMux "/2
  3/1 -> " 3 "/1
  " 3 "/1 -> " InputMux "/3

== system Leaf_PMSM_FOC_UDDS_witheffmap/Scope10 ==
  1 : Inport
  2 : Inport  Port=2
  " 1 " : DataTypeConversion
  " 2 " : DataTypeConversion
  " InputMux " : Mux  Inputs=2
  " S-Function " : S-Function  FunctionName=plecs  SFunctionDeploymentMode=off  EnableBusSupport=off
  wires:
  " InputMux "/1 -> " S-Function "/1
  1/1 -> " 1 "/1
  " 1 "/1 -> " InputMux "/1
  2/1 -> " 2 "/1
  " 2 "/1 -> " InputMux "/2

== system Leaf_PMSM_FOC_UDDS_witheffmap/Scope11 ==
  1 : Inport
  " InputMux " : Subsystem
  " S-Function " : S-Function  FunctionName=plecs  SFunctionDeploymentMode=off  EnableBusSupport=off
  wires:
  " InputMux "/1(Out) -> " S-Function "/1
  1/1 -> " InputMux "/1(In1)

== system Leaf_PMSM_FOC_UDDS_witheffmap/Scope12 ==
  1 : Inport
  " InputMux " : Subsystem
  " S-Function " : S-Function  FunctionName=plecs  SFunctionDeploymentMode=off  EnableBusSupport=off
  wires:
  " InputMux "/1(Out) -> " S-Function "/1
  1/1 -> " InputMux "/1(In1)

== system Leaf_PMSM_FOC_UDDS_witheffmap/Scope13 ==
  1 : Inport
  2 : Inport  Port=2
  " 1 " : DataTypeConversion
  " 2 " : DataTypeConversion
  " InputMux " : Mux  Inputs=2
  " S-Function " : S-Function  FunctionName=plecs  SFunctionDeploymentMode=off  EnableBusSupport=off
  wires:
  " InputMux "/1 -> " S-Function "/1
  1/1 -> " 1 "/1
  " 1 "/1 -> " InputMux "/1
  2/1 -> " 2 "/1
  " 2 "/1 -> " InputMux "/2

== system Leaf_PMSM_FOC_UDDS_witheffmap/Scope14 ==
  1 : Inport
  2 : Inport  Port=2
  3 : Inport  Port=3
  " 1 " : DataTypeConversion
  " 2 " : DataTypeConversion
  " 3 " : DataTypeConversion
  " InputMux " : Mux  Inputs=3
  " S-Function " : S-Function  FunctionName=plecs  SFunctionDeploymentMode=off  EnableBusSupport=off
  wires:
  " 3 "/1 -> " InputMux "/3
  3/1 -> " 3 "/1
  " 2 "/1 -> " InputMux "/2
  2/1 -> " 2 "/1
  " 1 "/1 -> " InputMux "/1
  1/1 -> " 1 "/1
  " InputMux "/1 -> " S-Function "/1

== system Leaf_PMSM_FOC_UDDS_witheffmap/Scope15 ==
  1 : Inport
  " InputMux " : Subsystem
  " S-Function " : S-Function  FunctionName=plecs  SFunctionDeploymentMode=off  EnableBusSupport=off
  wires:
  " InputMux "/1(Out) -> " S-Function "/1
  1/1 -> " InputMux "/1(In1)

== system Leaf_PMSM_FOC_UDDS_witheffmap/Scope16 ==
  1 : Inport
  " InputMux " : Subsystem
  " S-Function " : S-Function  FunctionName=plecs  SFunctionDeploymentMode=off  EnableBusSupport=off
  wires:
  1/1 -> " InputMux "/1(In1)
  " InputMux "/1(Out) -> " S-Function "/1

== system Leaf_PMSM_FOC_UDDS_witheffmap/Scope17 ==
  1 : Inport
  2 : Inport  Port=2
  " 1 " : DataTypeConversion
  " 2 " : DataTypeConversion
  " InputMux " : Mux  Inputs=2
  " S-Function " : S-Function  FunctionName=plecs  SFunctionDeploymentMode=off  EnableBusSupport=off
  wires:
  " InputMux "/1 -> " S-Function "/1
  1/1 -> " 1 "/1
  " 1 "/1 -> " InputMux "/1
  2/1 -> " 2 "/1
  " 2 "/1 -> " InputMux "/2

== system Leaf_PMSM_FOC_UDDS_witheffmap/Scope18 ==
  1 : Inport
  " InputMux " : Subsystem
  " S-Function " : S-Function  FunctionName=plecs  SFunctionDeploymentMode=off  EnableBusSupport=off
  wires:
  " InputMux "/1(Out) -> " S-Function "/1
  1/1 -> " InputMux "/1(In1)

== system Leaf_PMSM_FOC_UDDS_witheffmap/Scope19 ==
  1 : Inport
  " InputMux " : Subsystem
  " S-Function " : S-Function  FunctionName=plecs  SFunctionDeploymentMode=off  EnableBusSupport=off
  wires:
  1/1 -> " InputMux "/1(In1)
  " InputMux "/1(Out) -> " S-Function "/1

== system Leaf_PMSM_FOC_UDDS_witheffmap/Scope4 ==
  1 : Inport
  2 : Inport  Port=2
  " 1 " : DataTypeConversion
  " 2 " : DataTypeConversion
  " InputMux " : Mux  Inputs=2
  " S-Function " : S-Function  FunctionName=plecs  SFunctionDeploymentMode=off  EnableBusSupport=off
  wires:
  " InputMux "/1 -> " S-Function "/1
  1/1 -> " 1 "/1
  " 1 "/1 -> " InputMux "/1
  2/1 -> " 2 "/1
  " 2 "/1 -> " InputMux "/2

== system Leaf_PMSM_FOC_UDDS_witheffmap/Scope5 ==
  1 : Inport
  2 : Inport  Port=2
  " 1 " : DataTypeConversion
  " 2 " : DataTypeConversion
  " InputMux " : Mux  Inputs=2
  " S-Function " : S-Function  FunctionName=plecs  SFunctionDeploymentMode=off  EnableBusSupport=off
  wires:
  " InputMux "/1 -> " S-Function "/1
  1/1 -> " 1 "/1
  " 1 "/1 -> " InputMux "/1
  2/1 -> " 2 "/1
  " 2 "/1 -> " InputMux "/2

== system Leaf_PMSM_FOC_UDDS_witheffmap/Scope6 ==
  1 : Inport
  " 1 " : DataTypeConversion
  " InputMux " : Mux  Inputs=1
  " S-Function " : S-Function  FunctionName=plecs  SFunctionDeploymentMode=off  EnableBusSupport=off
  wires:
  " InputMux "/1 -> " S-Function "/1
  1/1 -> " 1 "/1
  " 1 "/1 -> " InputMux "/1

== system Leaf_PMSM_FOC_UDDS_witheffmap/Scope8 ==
  1 : Inport
  " InputMux " : Subsystem
  " S-Function " : S-Function  FunctionName=plecs  SFunctionDeploymentMode=off  EnableBusSupport=off
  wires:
  1/1 -> " InputMux "/1(In1)
  " InputMux "/1(Out) -> " S-Function "/1

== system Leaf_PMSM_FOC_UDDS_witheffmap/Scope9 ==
  1 : Inport
  " InputMux " : Subsystem
  " S-Function " : S-Function  FunctionName=plecs  SFunctionDeploymentMode=off  EnableBusSupport=off
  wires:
  1/1 -> " InputMux "/1(In1)
  " InputMux "/1(Out) -> " S-Function "/1

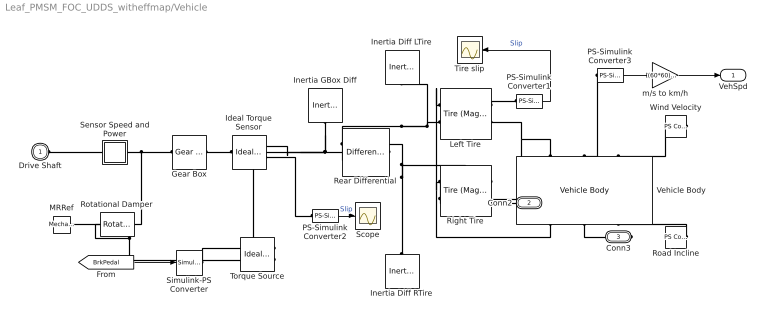
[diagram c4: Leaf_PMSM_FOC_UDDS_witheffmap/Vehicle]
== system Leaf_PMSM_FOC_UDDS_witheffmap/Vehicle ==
  Gear Box : fl_lib/Mechanical/Mechanisms/Gear Box  ratio=HEV_Param.Vehicle.Engine_Vehicle_Gear_Ratio  t_in_specify=off  t_in_priority=High  t_in=0 N*m  t_in_nominal_specify=off  t_in_nominal_unit=N*m  t_in_nominal_value=1  t_out_specify=off  t_out_priority=High  t_out=0 N*m  t_out_nominal_specify=off  t_out_nominal_unit=N*m  t_out_nominal_value=1
  Ideal Torque Sensor : fl_lib/Mechanical/Mechanical Sensors/Ideal Torque Sensor
  Inertia Diff LTire : fl_lib/Mechanical/Rotational Elements/Inertia  inertia=HEV_Param.Vehicle.Wheel_Inertia*2 kg*m^2  w_specify=on  w_priority=High  w=0 rad/s  w_nominal_specify=off  w_nominal_unit=rad/s  w_nominal_value=1  t_specify=off  t_priority=High  t=0 N*m  t_nominal_specify=off  t_nominal_unit=N*m  t_nominal_value=1
  Inertia Diff RTire : fl_lib/Mechanical/Rotational Elements/Inertia  inertia=HEV_Param.Vehicle.Wheel_Inertia*2 kg*m^2  w_specify=on  w_priority=High  w=0 rad/s  w_nominal_specify=off  w_nominal_unit=rad/s  w_nominal_value=1  t_specify=off  t_priority=High  t=0 N*m  t_nominal_specify=off  t_nominal_unit=N*m  t_nominal_value=1
  Inertia GBox Diff : fl_lib/Mechanical/Rotational Elements/Inertia  inertia=HEV_Param.Vehicle.Trans.Inertia kg*m^2  w_specify=on  w_priority=High  w=0 rad/s  w_nominal_specify=off  w_nominal_unit=rad/s  w_nominal_value=1  t_specify=off  t_priority=High  t=0 N*m  t_nominal_specify=off  t_nominal_unit=N*m  t_nominal_value=1
  Left Tire : sdl_lib/Tires & Vehicles/Tire (Magic Formula)  parameterization=1  F_z1=HEV_Param.Vehicle.Tire.Rated_Vertical_Load N  F_x1=HEV_Param.Vehicle.Tire.Rated_Peak_Long_Force N  kappa1=HEV_Param.Vehicle.Tire.Slip_At_Peak_Force  B_m=10  C_m=1.9  D_m=1  E_m=0.97  fz0=4e+3 N  p_Cx=1.685  p_Dx=[ 1.21 -0.037 ]  p_Ex=[ 0.344 0.095 -0.02 0 ]  p_Kx=[ 21.51 -0.163 0.245 ]  p_Hx=[ -0.002 0.002 ]  p_Vx=[ 0 0 ]  v_tr_thr=0.1 m/s  r_e=HEV_Param.Vehicle.Tire_Radius m  model_compliance=0  stiffness=1e+6 N/m  damping=1000 N/(m/s)  model_inertia=1  inertia=1e-2 kg*m^2  initial_velocity=0 rpm  model_resistance=1  resistance_model=1  coeff=0.015  p_tire=250e3 Pa  alpha=-0.003  beta=0.97  coeff_a=84e-4  coeff_b=6.2e-4 s/m  coeff_c=1.6e-4 s^2/m^2  v_thr=1e-3 m/s
  MRRef : fl_lib/Mechanical/Rotational Elements/Mechanical Rotational Reference
  PS-Simulink Converter1 : nesl_utility/PS-Simulink Converter  PhysicalDomain=network_engine_domain  SubClassName=ps_output  LeftPortType=input  RightPortType=output  PseudoPeriodic=off  Frequencies=[]  Unit=1  AffineConversion=off
  PS-Simulink Converter2 : nesl_utility/PS-Simulink Converter  PhysicalDomain=network_engine_domain  SubClassName=ps_output  LeftPortType=input  RightPortType=output  PseudoPeriodic=off  Frequencies=[]  Unit=1  AffineConversion=off
  PS-Simulink Converter3 : nesl_utility/PS-Simulink Converter  PhysicalDomain=network_engine_domain  SubClassName=ps_output  LeftPortType=input  RightPortType=output  PseudoPeriodic=off  Frequencies=[]  Unit=m/s  AffineConversion=off
  Rear Differential : sdl_lib/Gears/Differential  driveshaft_location=2  cd_ratio=1  friction_model=1  efficiency=[ 0.85 0.92 ]  mu_visc=[ 0 0 ] N*m/(rad/s)  pwr_thr=[ 0.001 0.001 ] W  carrier_inertia=0 kg*m^2  planet_inertia=0 kg*m^2  temperature_TLU=[ 280 300 320 ] K  efficiency_ss_TLU=[ 0.95 0.9 0.85 ]  efficiency_cd_TLU=[ 0.95 0.9 0.85 ]  thermal_mass=50 J/K  T_init=300 K
  Right Tire : sdl_lib/Tires & Vehicles/Tire (Magic Formula)  parameterization=1  F_z1=HEV_Param.Vehicle.Tire.Rated_Vertical_Load N  F_x1=HEV_Param.Vehicle.Tire.Rated_Peak_Long_Force N  kappa1=HEV_Param.Vehicle.Tire.Slip_At_Peak_Force  B_m=10  C_m=1.9  D_m=1  E_m=0.97  fz0=4e+3 N  p_Cx=1.685  p_Dx=[ 1.21 -0.037 ]  p_Ex=[ 0.344 0.095 -0.02 0 ]  p_Kx=[ 21.51 -0.163 0.245 ]  p_Hx=[ -0.002 0.002 ]  p_Vx=[ 0 0 ]  v_tr_thr=0.1 m/s  r_e=HEV_Param.Vehicle.Tire_Radius m  model_compliance=0  stiffness=1e+6 N/m  damping=1000 N/(m/s)  model_inertia=1  inertia=1e-2 kg*m^2  initial_velocity=0 rpm  model_resistance=1  resistance_model=1  coeff=0.015  p_tire=250e3 Pa  alpha=-0.003  beta=0.97  coeff_a=84e-4  coeff_b=6.2e-4 s/m  coeff_c=1.6e-4 s^2/m^2  v_thr=1e-3 m/s
  Road Incline : fl_lib/Physical Signals/Sources/PS Constant  constant=HEV_Param.Vehicle.Incline
  Rotational Damper : fl_lib/Mechanical/Rotational Elements/Rotational Damper  D=HEV_Param.Vehicle.Trans.Friction N*m/(rad/s)  w_specify=off  w_priority=High  w=0 rad/s  w_nominal_specify=off  w_nominal_unit=rad/s  w_nominal_value=1  t_specify=off  t_priority=High  t=0 N*m  t_nominal_specify=off  t_nominal_unit=N*m  t_nominal_value=1
  Scope : Scope
  Sensor Speed and Power : Subsystem
  Simulink-PS Converter : nesl_utility/Simulink-PS Converter  PhysicalDomain=network_engine_domain  SubClassName=ps_input  LeftPortType=input  RightPortType=output  PseudoPeriodic=off  Frequencies=[]  NoiseDistribution=none  NoiseParameters=[]  Unit=1  AffineConversion=off  FilteringAndDerivatives=zero  SimscapeFilterOrder=1  InputFilterTimeConstant=0.001  UdotUserProvided=1
  Tire slip : Scope
  Torque Source : fl_lib/Mechanical/Mechanical Sources/Ideal Torque Source
  Vehicle Body : sdl_lib/Tires & Vehicles/Vehicle Body  mass=HEV_Param.Vehicle.Mass kg  n_w=2  x_f=HEV_Param.Vehicle.Distance_CG_FrontAxle m  x_r=HEV_Param.Vehicle.Distance_CG_RearAxle m  y_c=HEV_Param.Vehicle.Distance_CG_Ground m  mass_var=simscape.enum.onoff.off  model_pitch=0  inertia=4000 kg*m^2  suspension_model=1  k_f=1e4 N/m  b_f=1e4 N/(m/s)  k_r=1e4 N/m  b_r=1e4 N/(m/s)  k_f_TLU=[-2000, -1000, 0, 1000, 2000] N  x_f_TLU=[-.4, -.2, 0, .2, .4] m  b_f_TLU=[-200, -100, 0, 100, 200] N  v_f_TLU=[-4, -2, 0, 2, 4] m/s  k_r_TLU=[-2000, -1000, 0, 1000, 2000] N  x_r_TLU=[-.4, -.2, 0, .2, .4] m  b_r_TLU=[-200, -100, 0, 100, 200] N  v_r_TLU=[-4, -2, 0, 2, 4] m/s  interp_method=simscape.enum.interpolation.linear  extrap_method=simscape.enum.extrapolation.linear  model_hardstop=0  upper_bound_f=.25 m  lower_bound_f=-.25 m  stop_k_f=1e6 N/m  stop_b_f=150 N/(m/s)  upper_bound_r=.25 m  lower_bound_r=-.25 m  stop_k_r=1e6 N/m  stop_b_r=150 N/(m/s)  initial_pitch=0 rad  initial_pitch_rate=0 rad/s  g=9.81 m/s^2  liftoff_warning=0  area=HEV_Param.Vehicle.Frontal_Area m^2  Cd=HEV_Param.Vehicle.Aero_Drag_Coeff  rho=1.18 kg/m^3  v_specify=on  v_priority=High  v=0 m/s  v_nominal_specify=off  v_nominal_unit=m/s  v_nominal_value=1
  Wind Velocity : fl_lib/Physical Signals/Sources/PS Constant  constant=0
  m/s to km/h : Gain  Gain=(60*60)/1000
  Drive Shaft : PMIOPort  Side=Left
  Conn2 : PMIOPort  Port=2  Side=Right
  Conn3 : PMIOPort  Port=3  Side=Right
  VehSpd : Outport
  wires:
  PS-Simulink Converter2/1 -> Scope/1  "Slip"
  PS-Simulink Converter3/1 -> m/s to km/h/1
  [BrkPedal] -> Simulink-PS Converter/1
  PS-Simulink Converter1/1 -> Tire slip/1  "Slip"
  m/s to km/h/1 -> VehSpd/1
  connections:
  Drive Shaft/RConn1 -- Sensor Speed and Power/LConn1
  Vehicle Body/LConn1 -- Right Tire/RConn2 -- Left Tire/RConn2
  Sensor Speed and Power/RConn1 -- Rotational Damper/LConn1 -- Gear Box/LConn1
  Torque Source/RConn2 -- Rotational Damper/RConn1 -- MRRef/LConn1
  Road Incline/RConn1 -- Vehicle Body/RConn3
  Inertia GBox Diff/LConn1 -- Rear Differential/LConn1 -- Torque Source/LConn1 -- Ideal Torque Sensor/RConn1
  Left Tire/RConn1 -- PS-Simulink Converter1/LConn1
  Wind Velocity/RConn1 -- Vehicle Body/LConn3
  Simulink-PS Converter/RConn1 -- Torque Source/RConn1
  PS-Simulink Converter2/LConn1 -- Ideal Torque Sensor/RConn2
  PS-Simulink Converter3/LConn1 -- Vehicle Body/LConn2
  Ideal Torque Sensor/LConn1 -- Gear Box/RConn1
  Vehicle Body/RConn1 -- Right Tire/LConn1 -- Left Tire/LConn1
  Vehicle Body/RConn2 -- Conn3/RConn1
  Left Tire/LConn2 -- Rear Differential/RConn2 -- Inertia Diff LTire/LConn1
  Right Tire/RConn1 -- Conn2/RConn1
  Rear Differential/RConn1 -- Right Tire/LConn2 -- Inertia Diff RTire/LConn1

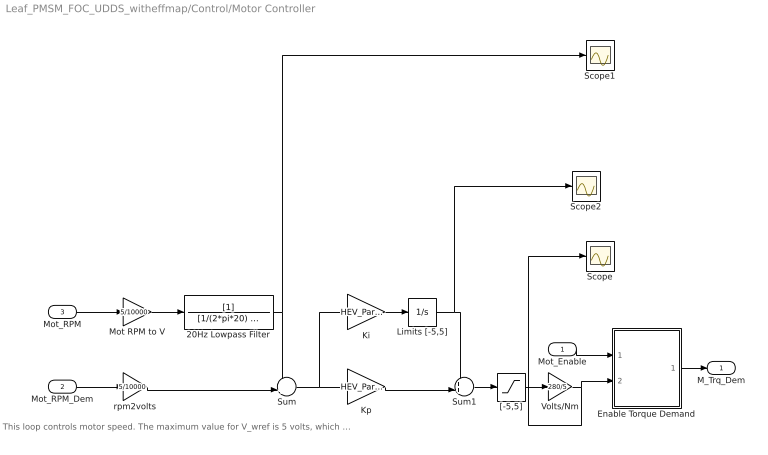
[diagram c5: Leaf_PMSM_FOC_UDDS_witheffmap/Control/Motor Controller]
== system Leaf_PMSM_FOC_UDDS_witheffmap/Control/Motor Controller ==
  note: This loop controls motor speed. The maximum value for V_wref is 5 volts, which is equivalent to a speed demand of 6500rpm.
  Mot_Enable : Inport
  Mot_RPM_Dem : Inport  Port=2
  Mot_RPM : Inport  Port=3
  20Hz Lowpass Filter : TransferFcn  Denominator=[1/(2*pi*20) 1]
  Enable Torque Demand : Subsystem
  Ki : Gain  Gain=HEV_Param.Control.Mot.Ki
  Kp : Gain  Gain=HEV_Param.Control.Mot.Kp
  Limits [-5,5] : Integrator  LimitOutput=on  UpperSaturationLimit=5  LowerSaturationLimit=-5
  Mot RPM to V : Gain  Gain=5/10000
  Scope : Scope
  Scope1 : Scope
  Scope2 : Scope
  Sum : Sum  Inputs=-+|
  Sum1 : Sum  Inputs=++|
  Volts/Nm : Gain  Gain=280/5
  "[-5,5]" : Saturate  UpperLimit=5  LowerLimit=-5
  rpm2volts : Gain  Gain=5/10000
  M_Trq_Dem : Outport
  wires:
  "[-5,5]"/1 -> Volts/Nm/1
  Mot_RPM/1 -> Mot RPM to V/1
  Sum1/1 -> "[-5,5]"/1
  Sum/1 -> Ki/1, Kp/1
  Ki/1 -> Limits [-5,5]/1
  Kp/1 -> Sum1/2
  Limits [-5,5]/1 -> Scope2/1, Sum1/1
  20Hz Lowpass Filter/1 -> Scope1/1, Sum/1
  rpm2volts/1 -> Sum/2
  Mot RPM to V/1 -> 20Hz Lowpass Filter/1
  Volts/Nm/1 -> Scope/1, Enable Torque Demand/2(TrqDemCtrl)
  Mot_RPM_Dem/1 -> rpm2volts/1
  Mot_Enable/1 -> Enable Torque Demand/1(Mot_Enable)
  Enable Torque Demand/1(TrqDem) -> M_Trq_Dem/1

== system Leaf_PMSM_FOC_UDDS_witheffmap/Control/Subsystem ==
  In1 : Inport
  Motor_RPM_Dem : Outport
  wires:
  In1/1 -> Motor_RPM_Dem/1

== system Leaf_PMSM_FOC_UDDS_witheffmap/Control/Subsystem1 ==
  In1 : Inport
  Accel : Outport
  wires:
  In1/1 -> Accel/1

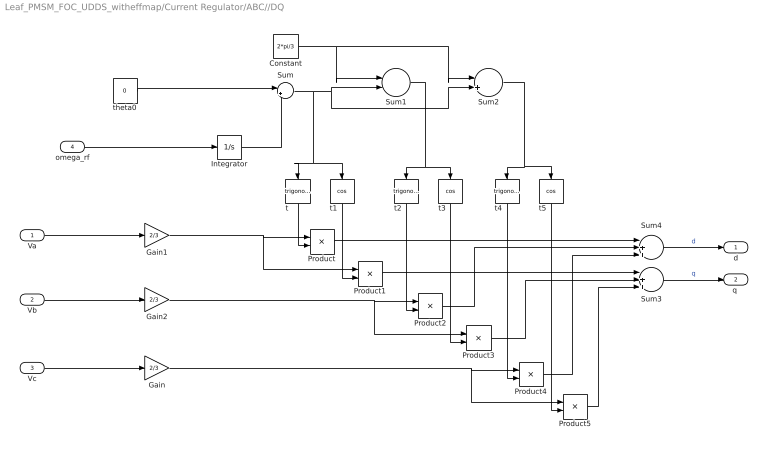
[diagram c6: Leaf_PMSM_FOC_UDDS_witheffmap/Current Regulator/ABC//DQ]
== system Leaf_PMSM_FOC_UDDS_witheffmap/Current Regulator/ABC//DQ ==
  Va : Inport
  Vb : Inport  Port=2
  Vc : Inport  Port=3
  omega_rf : Inport  Port=4
  Constant : Constant  Value=2*pi/3
  Gain : Gain  Gain=2/3
  Gain1 : Gain  Gain=2/3
  Gain2 : Gain  Gain=2/3
  Integrator : Integrator
  Product{,1..5} (6 alike) : Product
  Sum : Sum  Inputs=|++
  Sum1 : Sum  Inputs=|-+
  Sum2 : Sum  Inputs=|++
  Sum3 : Sum  Inputs=|+++
  Sum4 : Sum  Inputs=|+++
  t : Trigonometry
  t1 : Trigonometry  Operator=cos
  t2 : Trigonometry
  t3 : Trigonometry  Operator=cos
  t4 : Trigonometry
  t5 : Trigonometry  Operator=cos
  theta0 : Constant  Value=0
  d : Outport
  "q " : Outport  Port=2
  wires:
  theta0/1 -> Sum/1
  Sum/1 -> t1/1, t/1, Sum2/2, Sum1/2
  Sum2/1 -> t5/1, t4/1
  Integrator/1 -> Sum/2
  t4/1 -> Product4/2
  Sum1/1 -> t2/1, t3/1
  Product/1 -> Sum4/1
  t/1 -> Product/2
  Va/1 -> Gain1/1
  Constant/1 -> Sum1/1, Sum2/1
  Vc/1 -> Gain/1
  Product3/1 -> Sum3/2
  Gain2/1 -> Product3/1, Product2/1
  t5/1 -> Product5/2
  t1/1 -> Product1/2
  Gain/1 -> Product5/1, Product4/1
  Product1/1 -> Sum3/1
  Gain1/1 -> Product1/1, Product/1
  Product5/1 -> Sum3/3
  Product2/1 -> Sum4/2
  Product4/1 -> Sum4/3
  Vb/1 -> Gain2/1
  t3/1 -> Product3/2
  t2/1 -> Product2/2
  Sum4/1 -> d/1  "d"
  Sum3/1 -> "q "/1  "q"
  omega_rf/1 -> Integrator/1

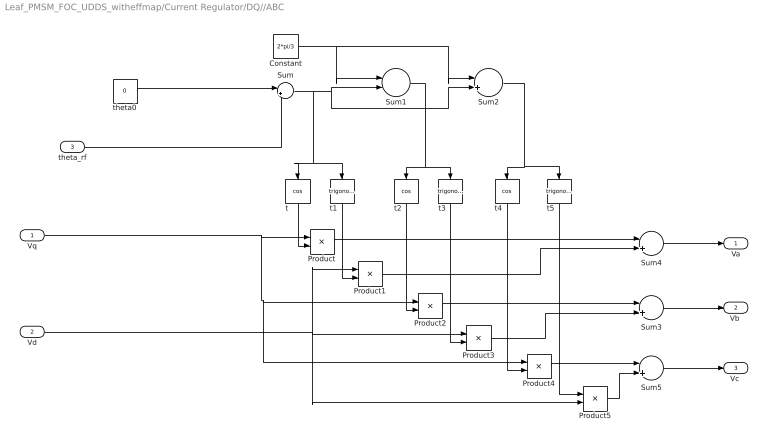
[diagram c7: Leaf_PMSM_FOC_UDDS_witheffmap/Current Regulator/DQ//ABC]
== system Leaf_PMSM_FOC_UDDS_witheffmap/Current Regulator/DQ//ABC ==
  Vq : Inport
  Vd : Inport  Port=2
  theta_rf : Inport  Port=3
  Constant : Constant  Value=2*pi/3
  Product{,1..5} (6 alike) : Product
  Sum{,2..5} (5 alike) : Sum  Inputs=|++
  Sum1 : Sum  Inputs=|-+
  t : Trigonometry  Operator=cos
  t1 : Trigonometry
  t2 : Trigonometry  Operator=cos
  t3 : Trigonometry
  t4 : Trigonometry  Operator=cos
  t5 : Trigonometry
  theta0 : Constant  Value=0
  Va : Outport
  "Vb " : Outport  Port=2
  "Vc " : Outport  Port=3
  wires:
  theta0/1 -> Sum/1
  Sum/1 -> t1/1, t/1, Sum2/2, Sum1/2
  Sum2/1 -> t5/1, t4/1
  Sum1/1 -> t2/1, t3/1
  t/1 -> Product/2
  Constant/1 -> Sum1/1, Sum2/1
  Product3/1 -> Sum3/2
  t1/1 -> Product1/2
  t3/1 -> Product3/2
  t2/1 -> Product2/2
  Sum4/1 -> Va/1
  Sum3/1 -> "Vb "/1
  theta_rf/1 -> Sum/2
  Vd/1 -> Product5/2, Product1/1, Product3/1
  Product/1 -> Sum4/1
  Product1/1 -> Sum4/2
  Product2/1 -> Sum3/1
  Vq/1 -> Product4/1, Product2/1, Product/1
  t4/1 -> Product4/2
  t5/1 -> Product5/1
  Product4/1 -> Sum5/1
  Product5/1 -> Sum5/2
  Sum5/1 -> "Vc "/1
